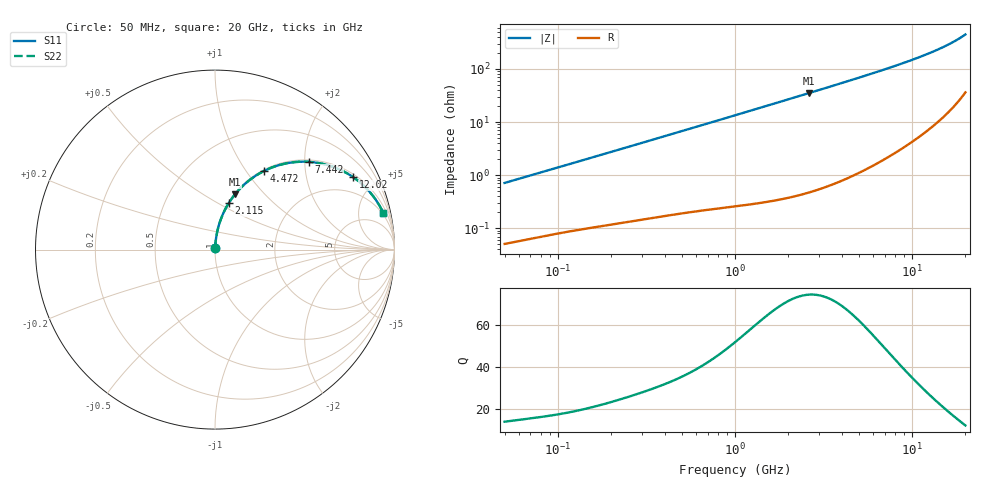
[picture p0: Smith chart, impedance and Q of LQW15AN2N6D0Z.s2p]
!Murata Part Number: LQW15AN2N6D0Z
!These Parameters are Measured in Series Mode Connection
!  o--[Z]--o
!Port1  Port2
!  o-------o
!Freq. Start=50[MHz] Stop=20[GHz], 401[Steps]
# Hz S RI R 50
!Freq.(Hz) S11(Real) S11(Imag) S21(Real) S21(Imag) S12(Real) S12(Imag) S22(Real) S22(Imag)
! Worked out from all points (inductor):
!   401 points, 50 MHz to 20 GHz, reference 50 ohm
!   read as one part in series: L = 2.25 nH near 51.52 MHz
!   highest Q = 74.3 at 2.608 GHz (marker M1), where L = 2.13 nH
!   S11 on the Smith chart (normalised r, x): 50 MHz: 1.00, +0.01; 2.115 GHz: 1.01, +0.56; 4.472 GHz: 1.02, +1.21; 7.442 GHz: 1.05, +2.09; 12.02 GHz: 1.13, +3.73; 20 GHz: 1.72, +8.85
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5e7  0.000558 0.00711  0.9994 -0.00711  0.9994 -0.00711  0.000558 0.00711
1.364002e8  0.00131 0.0188  0.9987 -0.0188  0.9987 -0.0188  0.00131 0.0188
3.721004e8  0.00414 0.05  0.9959 -0.05  0.9959 -0.05  0.00414 0.05
6.285508e8  0.00912 0.0833  0.9909 -0.0833  0.9909 -0.0833  0.00912 0.0833
1e9  0.02 0.1305  0.98 -0.1305  0.98 -0.1305  0.02 0.1305
1.521052e9  0.0423 0.1936  0.9577 -0.1936  0.9577 -0.1936  0.0423 0.1936
2.114743e9  0.0769 0.2596  0.9231 -0.2596  0.9231 -0.2596  0.0769 0.2596
2.608132e9  0.1118 0.3084  0.8882 -0.3084  0.8882 -0.3084  0.1118 0.3084
2.728004e9  0.1209 0.3194  0.8791 -0.3194  0.8791 -0.3194  0.1209 0.3194
3.519108e9  0.1864 0.3825  0.8136 -0.3825  0.8136 -0.3825  0.1864 0.3825
4.472136e9  0.2717 0.4373  0.7283 -0.4373  0.7283 -0.4373  0.2717 0.4373
5.856089e9  0.3952 0.4801  0.6048 -0.4801  0.6048 -0.4801  0.3952 0.4801
6.601595e9  0.4574 0.4885  0.5426 -0.4885  0.5426 -0.4885  0.4574 0.4885
7.442007e9  0.5221 0.4889  0.4779 -0.4889  0.4779 -0.4889  0.5221 0.4889
8.389408e9  0.5875 0.4804  0.4125 -0.4804  0.4125 -0.4804  0.5875 0.4804
9.457416e9  0.6517 0.4631  0.3483 -0.4631  0.3483 -0.4631  0.6517 0.4631
1.201863e10  0.7691 0.4041  0.2309 -0.4041  0.2309 -0.4041  0.7691 0.4041
1.375312e10  0.8254 0.3591  0.1746 -0.3591  0.1746 -0.3591  0.8254 0.3591
1.573793e10  0.8733 0.3078  0.1267 -0.3078  0.1267 -0.3078  0.8733 0.3078
1.747767e10  0.9044 0.2647  0.0956 -0.2647  0.0956 -0.2647  0.9044 0.2647
1.940974e10  0.9301 0.2197  0.0699 -0.2197  0.0699 -0.2197  0.9301 0.2197
2e10  0.9364 0.2065  0.0636 -0.2065  0.0636 -0.2065  0.9364 0.2065
